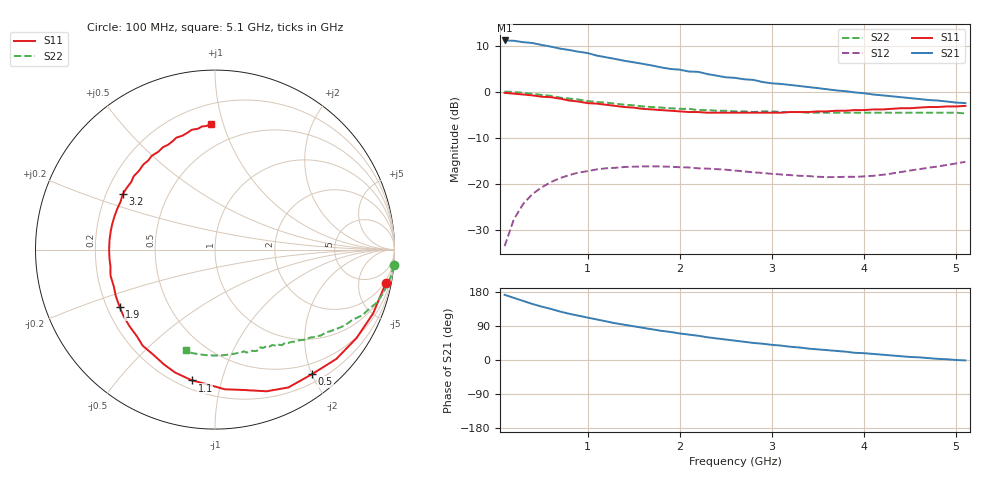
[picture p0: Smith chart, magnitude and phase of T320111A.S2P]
!AT-32011
!S and NOISE PARAMETERS at Vce=1 V  Ic=1mA.  LAST UPDATED 01-05-95
# ghz s ma r 50
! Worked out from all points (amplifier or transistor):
!   51 points, 100 MHz to 5.1 GHz, reference 50 ohm
!   highest |S21| = 11.1 dB at 100 MHz (marker M1)
!   |S21| within 3 dB of that: start of sweep to 1.048 GHz
!   unconditionally stable (mu >= 1): 2.759 GHz to end of sweep
!   at 900 MHz: K = 0.29, MSG = 13.1 dB, |S12| = -17.6 dB
!   at 2.6 GHz: K = 0.93, MSG = 10.1 dB, |S12| = -17.1 dB
!   at 5.1 GHz: K = 1.10, MAG = 4.5 dB, |S12| = -15.2 dB
!   lowest NFmin = 0.42 dB at 500 MHz
!   S11 on the Smith chart (normalised r, x): 100 MHz: 2, -10; 500 MHz: 0.33, -2.01; 1.1 GHz: 0.25, -0.81; 1.9 GHz: 0.25, -0.26; 3.2 GHz: 0.27, +0.26; 5.1 GHz: 0.33, +0.91
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0.1  0.97 -11.0  3.59 172.0  0.021 83.0  1 -5.0
0.2  0.95 -22.0  3.56 164.0  0.041 77.0  0.99 -9.0
0.4  0.91 -42.0  3.37 148.0  0.077 64.0  0.95 -18.0
0.5  0.88 -52.0  3.21 141.0  0.091 59.0  0.92 -21.0
0.6  0.87 -62.0  3.08 135.0  0.104 54.0  0.9 -24.0
0.7  0.84 -70.0  2.93 128.0  0.115 49.0  0.86 -27.0
0.8  0.8 -78.0  2.83 122.0  0.124 44.0  0.84 -30.0
1  0.75 -94.0  2.62 112.0  0.137 37.0  0.79 -35.0
1.1  0.74 -100.0  2.46 107.0  0.143 34.0  0.77 -37.0
1.3  0.7 -114.0  2.26 97.0  0.149 28.0  0.74 -41.0
1.4  0.68 -120.0  2.16 93.0  0.152 25.0  0.72 -43.0
1.8  0.63 -144.0  1.83 77.0  0.154 16.0  0.67 -50.0
1.9  0.62 -149.0  1.76 74.0  0.153 15.0  0.66 -52.0
2.2  0.6 -166.0  1.64 64.0  0.147 11.0  0.63 -57.0
2.3  0.59 -171.0  1.55 60.0  0.146 10.0  0.63 -58.0
2.6  0.59 175.0  1.41 51.0  0.139 8.0  0.61 -62.0
2.8  0.59 166.0  1.34 45.0  0.133 8.0  0.6 -65.0
3.2  0.6 149.0  1.18 35.0  0.124 10.0  0.6 -71.0
3.5  0.61 138.0  1.09 28.0  0.119 14.0  0.59 -76.0
3.9  0.63 124.0  0.98 19.0  0.119 21.0  0.59 -82.0
4.3  0.65 111.0  0.89 12.0  0.129 30.0  0.59 -89.0
5.1  0.7 92.0  0.75 -1.0  0.173 35.0  0.58 -106.0
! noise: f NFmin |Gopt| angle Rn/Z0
0.5  0.42  0.79  26  0.44
0.9  0.71  0.7  54  0.35
1.8  1.37  0.53  119  0.18
2.4  1.8  0.55  158  0.08
